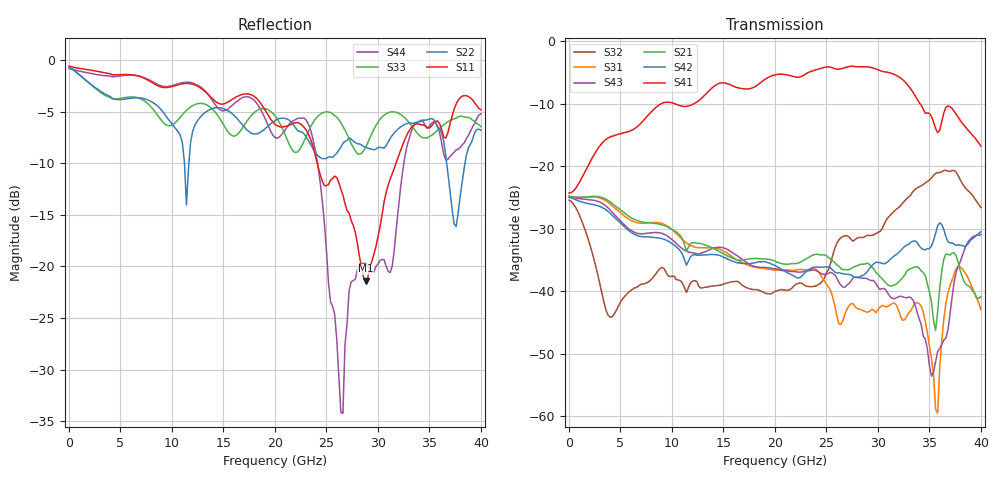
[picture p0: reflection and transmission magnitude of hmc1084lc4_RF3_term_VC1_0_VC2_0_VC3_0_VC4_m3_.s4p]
!Agilent Technologies,N5224A,MY51441122,A.09.40.06
!Agilent N5224A: A.09.40.06
!Date: Thursday, June 19, 2014 00:51:35
!Correction: S11(Full 4 Port(1,2,3,4))
!S12(Full 4 Port(1,2,3,4))
!S13(Full 4 Port(1,2,3,4))
!S14(Full 4 Port(1,2,3,4))
!S21(Full 4 Port(1,2,3,4))
!S22(Full 4 Port(1,2,3,4))
!S23(Full 4 Port(1,2,3,4))
!S24(Full 4 Port(1,2,3,4))
!S31(Full 4 Port(1,2,3,4))
!S32(Full 4 Port(1,2,3,4))
!S33(Full 4 Port(1,2,3,4))
!S34(Full 4 Port(1,2,3,4))
!S41(Full 4 Port(1,2,3,4))
!S42(Full 4 Port(1,2,3,4))
!S43(Full 4 Port(1,2,3,4))
!S44(Full 4 Port(1,2,3,4))
!S4P File: Measurements: <S11,S12,S13,S14>,
!<S21,S22,S23,S24>,
!<S31,S32,S33,S34>,
!<S41,S42,S43,S44>:
# Hz S  dB  R 50
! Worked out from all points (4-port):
!   201 points, 10 MHz to 40 GHz, reference 50 ohm
!   strongest paths, dB at 10 MHz, 10.01 GHz, 20 GHz, 30 GHz, 40 GHz:
!     S41: -24.3, -9.8, -5.4, -4.5, -16.8
!     S42: -25.0, -32.4, -35.9, -35.4, -30.5
!     S21: -24.8, -30.1, -35.2, -37.3, -40.9
!     S43: -24.8, -31.7, -36.4, -39.3, -30.9
!     S31: -24.8, -30.1, -36.6, -42.9, -42.9
!     S32: -25.4, -37.6, -40.0, -30.6, -26.6
!   lowest |S11| = -21.4 dB at 28.8 GHz (marker M1), VSWR 1.19, Z = 48 - j8.13 ohm
!   |S11| at or under -10 dB: 24.1 GHz to 31.76 GHz (7.657 GHz wide, 27.4 % of centre)
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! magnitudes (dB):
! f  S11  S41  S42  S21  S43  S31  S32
! 10 MHz  -0.6  -24.3  -25.0  -24.8  -24.8  -24.8  -25.4
! 4.009 GHz  -1.3  -15.3  -27.5  -25.7  -27.0  -26.0  -44.1
! 23 GHz  -6.8  -5.2  -36.9  -34.9  -36.7  -36.6  -39.2
! 26.4 GHz  -12.5  -4.4  -37.1  -36.3  -39.0  -45.3  -31.5
! 28.8 GHz  -21.4  -4.1  -37.1  -35.6  -37.9  -43.3  -31.2
! 35.4 GHz  -6.1  -12.9  -31.9  -44.7  -53.0  -53.3  -21.5
! 40 GHz  -4.8  -16.8  -30.5  -40.9  -30.9  -42.9  -26.6
